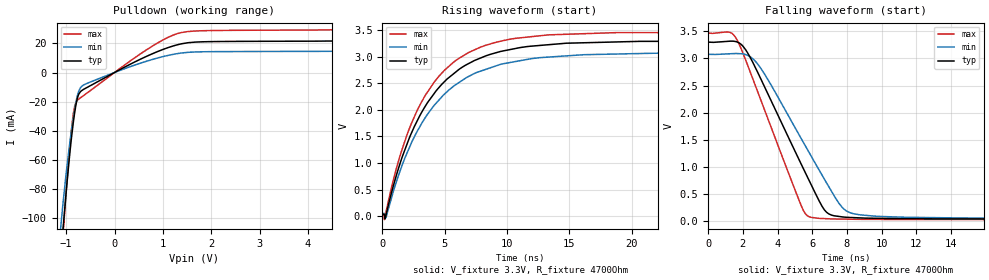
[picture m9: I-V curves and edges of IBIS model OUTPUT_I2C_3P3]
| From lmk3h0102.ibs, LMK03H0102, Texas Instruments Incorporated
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[Model]   OUTPUT_I2C_3P3
Model_type   Open_drain
Polarity   Non-Inverting
Vmeas = 1.65
Vref = 3.3
Cref = 10pF
Rref = 4700
|   typ   min   max
C_comp   0.7pF   0.5pF   0.9pF
[Voltage Range]   3.3   3.135   3.465
[Temperature Range]   45   125   -40
[Pullup Reference]   3.3   3.135   3.465
[Pulldown Reference]   0   0   0
[Power Clamp Reference]   3.3   3.135   3.465
[GND Clamp Reference]   0   0   0
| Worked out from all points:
|   slope of the pulldown table from 0 to 0.495 V, typ, clamps not added: 58.3 ohm
|   falling waveform, V_fixture 3.3V, R_fixture 4700Ohm: 20-80 % time 2.91ns typ, 3.22ns min, 2.45ns max; typ from 3.3 V to 0.038 V
|   rising waveform, V_fixture 3.3V, R_fixture 4700Ohm: 20-80 % time 4.52ns typ, 4.73ns min, 4.22ns max; typ from 0.038 V to 3.3 V
[Pulldown]
|   Voltage   I(typ)   I(min)   I(max)
-3.3V     -1.111A    -994.6mA   -1.235A
-1.181V   -155mA     -130.2mA   -166mA
-1.063V   -106.3mA   -88.93mA   -110.1mA
-1.013V   -87.04mA   -73.2mA    -87.67mA
-914.1mV  -52.02mA   -45.46mA   -46.91mA
-854.7mV  -34.77mA   -31.34mA   -28.74mA
-795.3mV  -21.66mA   -19.82mA   -20.37mA
-735.9mV  -14.64mA   -12.47mA   -18.18mA
16.5mV    299uA      212.7uA    413.8uA
1.214V    18.26mA    12.49mA    25.72mA
1.828V    21.11mA    14.25mA    28.71mA
6.6V      22.24mA    14.99mA    30.18mA
[Ramp]
R_load = 4700
|   typ   min   max
dV/dt_r   1.95697/4.49446e-09   1.815/4.72719e-09   2.06149/4.20764e-09
dV/dt_f   1.95697/2.91183e-09   1.81491/3.21923e-09   2.06149/2.44626e-09
[Falling Waveform]
V_fixture = 3.3V
V_fixture_min = 3.135V
V_fixture_max = 3.465V
R_fixture = 4700Ohm
C_fixture = 0F
|   Time   V(typ)   V(min)   V(max)
0s        3.3V       3.076V     3.465V
1.246ns   3.317V     3.085V     3.482V
1.686ns   3.3V       3.09V      3.329V
2.165ns   3.157V     3.07V      2.968V
2.909ns   2.708V     2.874V     2.341V
5.613ns   886.3mV    1.382V     133.2mV
6.822ns   165.8mV    707.1mV    47.42mV
7.756ns   79.48mV    244.5mV    40.04mV
8.697ns   62.89mV    120.9mV    35.86mV
1.25us    38.38mV    51.11mV    29.18mV
[Rising Waveform]
V_fixture = 3.3V
V_fixture_min = 3.135V
V_fixture_max = 3.465V
R_fixture = 4700Ohm
C_fixture = 0F
|   Time   V(typ)   V(min)   V(max)
0s        38.38mV    51.11mV    29.18mV
167.6ps   28.86mV    50.85mV    -65.19mV
287.3ps   13.49mV    -28.23mV   67.63mV
1.373ns   955.3mV    817.8mV    1.1V
2.718ns   1.756V     1.562V     1.95V
4.164ns   2.309V     2.087V     2.524V
5.708ns   2.677V     2.444V     2.896V
11.05ns   3.171V     2.925V     3.354V
18.82ns   3.278V     3.05V      3.453V
1.25us    3.3V       3.076V     3.465V
